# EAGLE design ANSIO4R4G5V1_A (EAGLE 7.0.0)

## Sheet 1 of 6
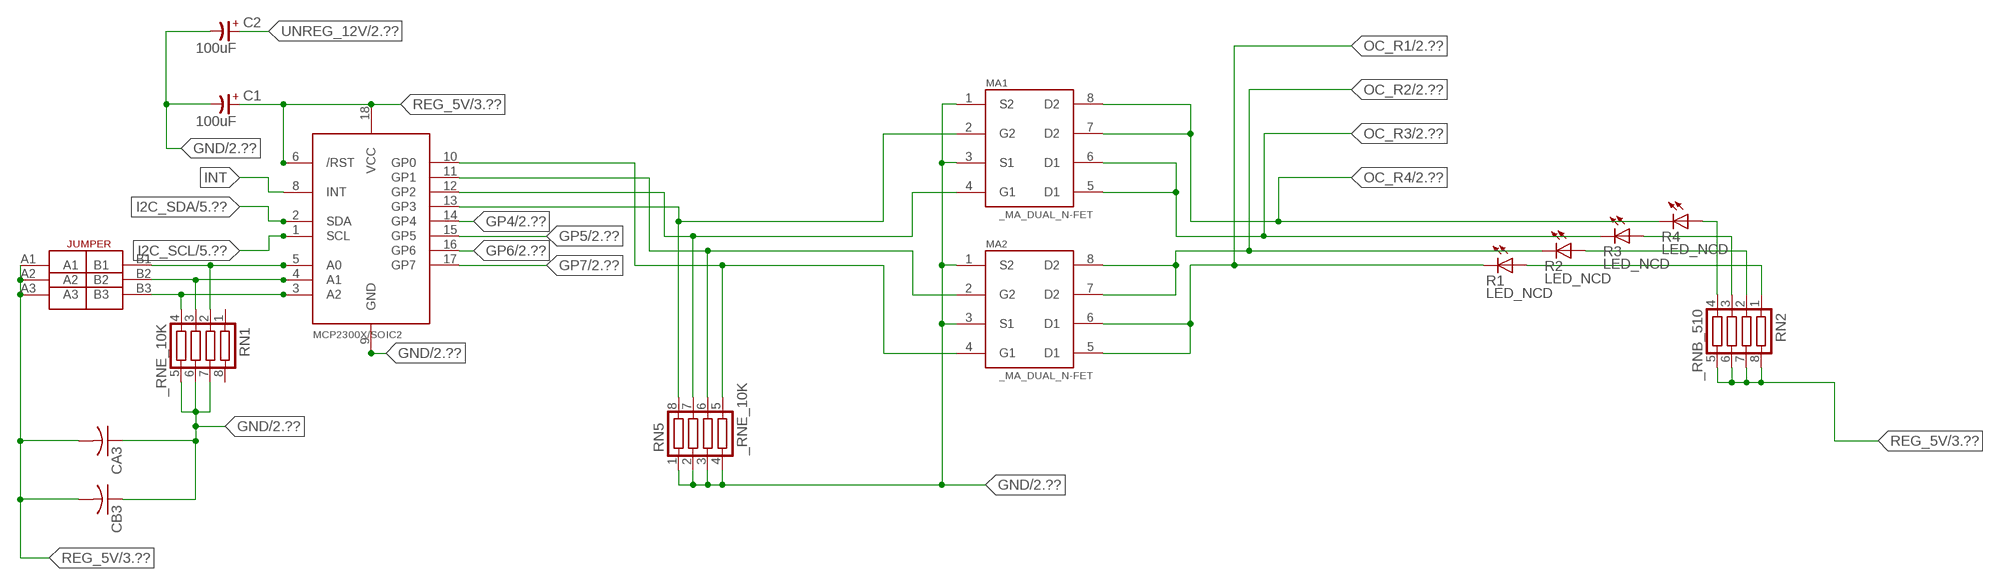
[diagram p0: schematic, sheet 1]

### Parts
C1  100uF  CP-E-025X060  [E-025X060]
C2  100uF  CP-E-025X060  [E-025X060]
CA3  CC1206KRX7R9BB104C1206K  [CC1206KRX7R9BB104]
CB3  TMK316F106ZL-TC1206K  [TMK316F106ZL-T]
IC2  MCP2300X/SO  [SO18W]
MA1  _MA_DUAL_N-FET  [_MA_DUAL_N-FET]
MA2  _MA_DUAL_N-FET  [_MA_DUAL_N-FET]
R1  LED_NCD  [CHIPLED_0603]
R2  LED_NCD  [CHIPLED_0603]
R3  LED_NCD  [CHIPLED_0603]
R4  LED_NCD  [CHIPLED_0603]
RN1  _RNE_10K  [RNE]
RN2  _RNB_510  [RNB]
RN5  _RNE_10K  [RNE]
U$18  JUMPER_3X2  [JUMPER_3X2]

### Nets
GND: C1.- C2.- CA3.1 CB3.1 IC2.9(GND) MA1.1(S2) MA1.3(S1) MA2.1(S2) MA2.3(S1) RN1.5 RN1.6 RN1.7 RN5.1 RN5.2 RN5.3 RN5.4 ; also sheet 2,3,4,5,6
GP4: IC2.14(GP4) ; also sheet 2
GP5: IC2.15(GP5) ; also sheet 2
GP6: IC2.16(GP6) ; also sheet 2
GP7: IC2.17(GP7) ; also sheet 2
I2C_SCL: IC2.1(SCL) ; also sheet 5,6
I2C_SDA: IC2.2(SDA) ; also sheet 5,6
INT: IC2.8(INT)
N$6: IC2.5(A0) RN1.2 U$18.B1
N$7: IC2.4(A1) RN1.3 U$18.B2
N$8: IC2.3(A2) RN1.4 U$18.B3
N$20: IC2.13(GP3) MA1.2(G2) RN5.8
N$21: IC2.12(GP2) MA1.4(G1) RN5.7
N$22: IC2.11(GP1) MA2.2(G2) RN5.6
N$23: IC2.10(GP0) MA2.4(G1) RN5.5
N$29: R4.A RN2.4
N$30: R3.A RN2.3
N$31: R2.A RN2.2
N$32: R1.A RN2.1
OC_R1: MA2.5(D1) MA2.6(D1) R1.C ; also sheet 2
OC_R2: MA2.7(D2) MA2.8(D2) R2.C ; also sheet 2
OC_R3: MA1.5(D1) MA1.6(D1) R3.C ; also sheet 2
OC_R4: MA1.7(D2) MA1.8(D2) R4.C ; also sheet 2
REG_5V: C1.+ CA3.2 CB3.2 IC2.6(/RST) IC2.18(VCC) RN2.5 RN2.6 RN2.7 RN2.8 U$18.A1 U$18.A2 U$18.A3 ; also sheet 3,4,5,6
UNREG_12V: C2.+ ; also sheet 2,3
Unconnected: RN1.1 RN1.8

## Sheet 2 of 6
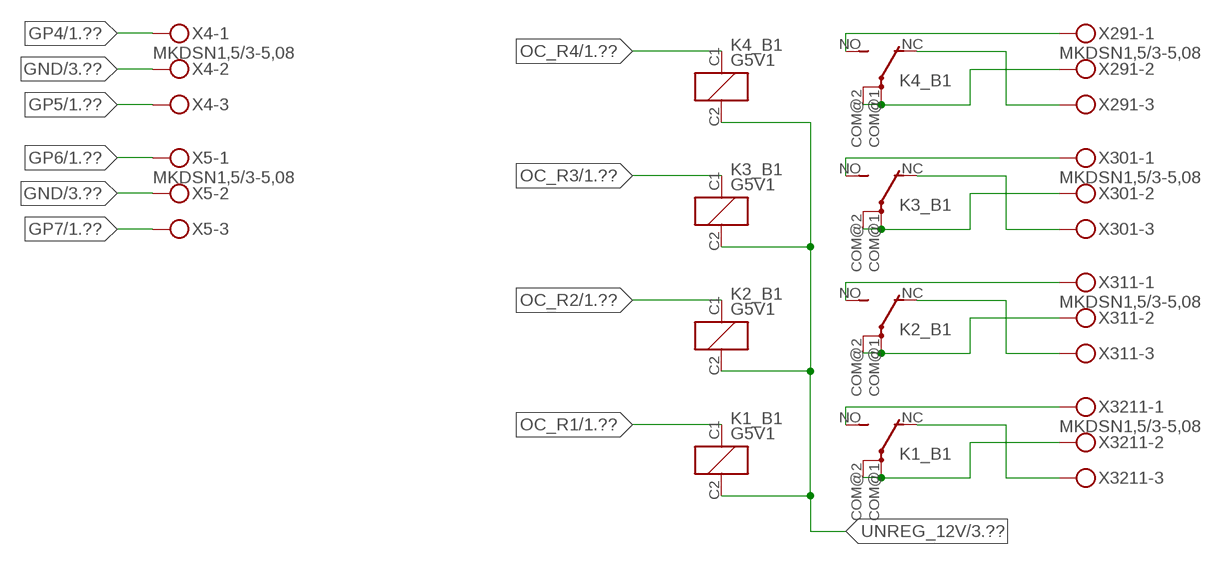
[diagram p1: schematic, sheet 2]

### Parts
K1_B1  G5V1  [G5V1]
K2_B1  G5V1  [G5V1]
K3_B1  G5V1  [G5V1]
K4_B1  G5V1  [G5V1]
X4  MKDSN1,5/3-5,08  [MKDSN1,5/3-5,08]
X5  MKDSN1,5/3-5,08  [MKDSN1,5/3-5,08]
X291  MKDSN1,5/3-5,08  [MKDSN1,5/3-5,08]
X301  MKDSN1,5/3-5,08  [MKDSN1,5/3-5,08]
X311  MKDSN1,5/3-5,08  [MKDSN1,5/3-5,08]
X3211  MKDSN1,5/3-5,08  [MKDSN1,5/3-5,08]

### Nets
GND: X4.2 X5.2 ; also sheet 1,3,4,5,6
GP4: X4.1 ; also sheet 1
GP5: X4.3 ; also sheet 1
GP6: X5.1 ; also sheet 1
GP7: X5.3 ; also sheet 1
N$215: K4_B1.NO(2:S) X291.1
N$216: K4_B1.NC(2:O) X291.3
N$217: K4_B1.COM@1(2:P) K4_B1.COM@2(2:P) X291.2
N$218: K3_B1.NO(2:S) X301.1
N$219: K3_B1.NC(2:O) X301.3
N$220: K3_B1.COM@1(2:P) K3_B1.COM@2(2:P) X301.2
N$221: K2_B1.NO(2:S) X311.1
N$222: K2_B1.NC(2:O) X311.3
N$223: K2_B1.COM@1(2:P) K2_B1.COM@2(2:P) X311.2
N$224: K1_B1.NO(2:S) X3211.1
N$225: K1_B1.NC(2:O) X3211.3
N$226: K1_B1.COM@1(2:P) K1_B1.COM@2(2:P) X3211.2
OC_R1: K1_B1.C1(1:C1) ; also sheet 1
OC_R2: K2_B1.C1(1:C1) ; also sheet 1
OC_R3: K3_B1.C1(1:C1) ; also sheet 1
OC_R4: K4_B1.C1(1:C1) ; also sheet 1
UNREG_12V: K1_B1.C2(1:C2) K2_B1.C2(1:C2) K3_B1.C2(1:C2) K4_B1.C2(1:C2) ; also sheet 1,3

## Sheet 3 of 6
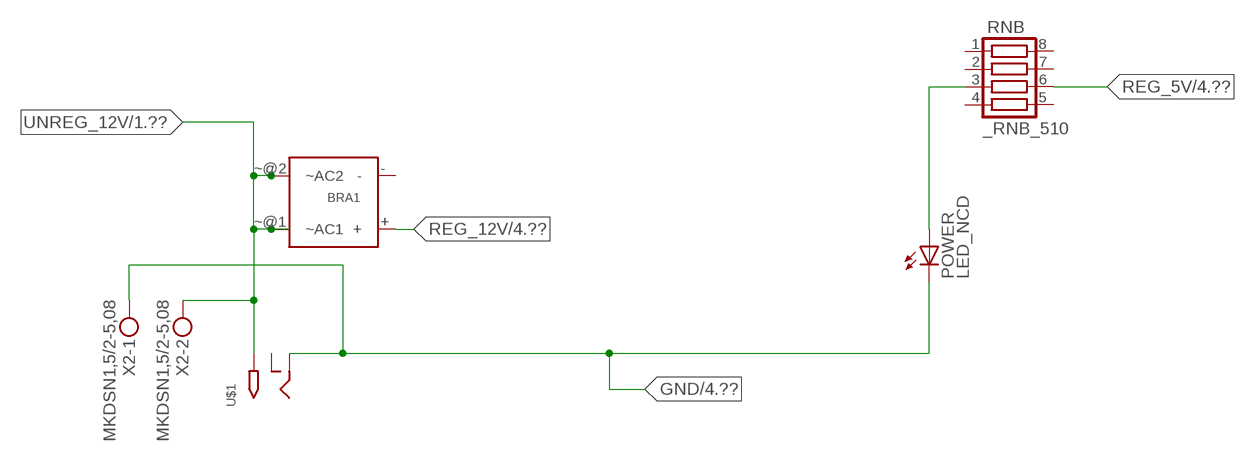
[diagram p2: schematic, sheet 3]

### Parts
BRA1  MB2S_  [MB2S]
POWER  LED_NCD  [CHIPLED_0603]
RNB  _RNB_510  [RNB]
U$1  2.1MMJACK  [PJ-102A]
X2  MKDSN1,5/2-5,08  [MKDSN1,5/2-5,08]

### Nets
GND: POWER.C U$1.RING X2.1 ; also sheet 1,2,4,5,6
N$2: POWER.A RNB.3
REG_5V: RNB.6 ; also sheet 1,4,5,6
REG_12V: BRA1.+ ; also sheet 4
UNREG_12V: BRA1.~@1(~AC1) BRA1.~@2(~AC2) U$1.TIP X2.2 ; also sheet 1,2
Unconnected: BRA1.- RNB.1 RNB.2 RNB.4 RNB.5 RNB.7 RNB.8 U$1.RING_SW

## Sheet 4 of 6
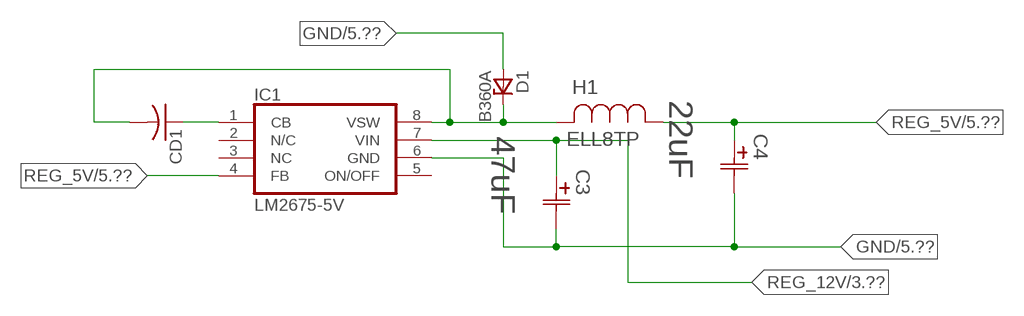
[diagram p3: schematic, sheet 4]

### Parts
C3  47uF  490-5463-6-NDCAP  [C2917(7343)-Y]
C4  22uF  490-5463-6-NDCAP  [C2917(7343)-Y]
CD1  _CD_10NF_50VC1206K  [_CD_10NF_50V]
D1  B360A  [DO214AC_ZENER]
H1  ELL8TP  [IND_ELL8TP]
IC1  LM2675-5V  LM2675  [SO-8]

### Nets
GND: C3.2(C2) C4.2(C2) D1.A IC1.6(GND) ; also sheet 1,2,3,5,6
N$1: CD1.2 D1.C H1.2 IC1.8(VSW)
N$3: CD1.1 IC1.1(CB)
REG_5V: C4.1(C1) H1.1 IC1.4(FB) ; also sheet 1,3,5,6
REG_12V: C3.1(C1) IC1.7(VIN) ; also sheet 3
Unconnected: IC1.2(N/C) IC1.5(ON/OFF)

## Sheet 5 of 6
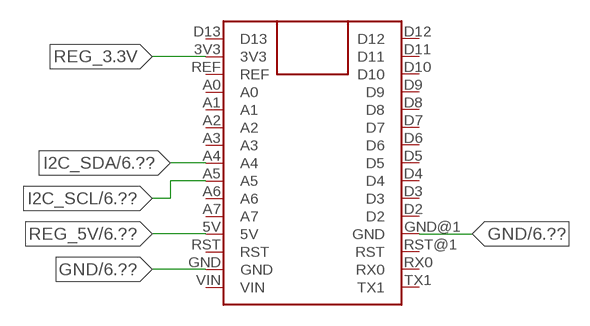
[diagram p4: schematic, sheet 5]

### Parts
FOR_NANO  ARDUINO_NANO  [ARDUINO_NANO]

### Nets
GND: FOR_NANO.GND FOR_NANO.GND@1(GND) ; also sheet 1,2,3,4,6
I2C_SCL: FOR_NANO.A5 ; also sheet 1,6
I2C_SDA: FOR_NANO.A4 ; also sheet 1,6
REG_3.3V: FOR_NANO.3V3
REG_5V: FOR_NANO.5V ; also sheet 1,3,4,6
Unconnected: FOR_NANO.A0 FOR_NANO.A1 FOR_NANO.A2 FOR_NANO.A3 FOR_NANO.A6 FOR_NANO.A7 FOR_NANO.D2 FOR_NANO.D3 FOR_NANO.D4 FOR_NANO.D5 FOR_NANO.D6 FOR_NANO.D7 FOR_NANO.D8 FOR_NANO.D9 FOR_NANO.D10 FOR_NANO.D11 FOR_NANO.D12 FOR_NANO.D13 FOR_NANO.REF FOR_NANO.RST FOR_NANO.RST@1(RST) FOR_NANO.RX0 FOR_NANO.TX1 FOR_NANO.VIN

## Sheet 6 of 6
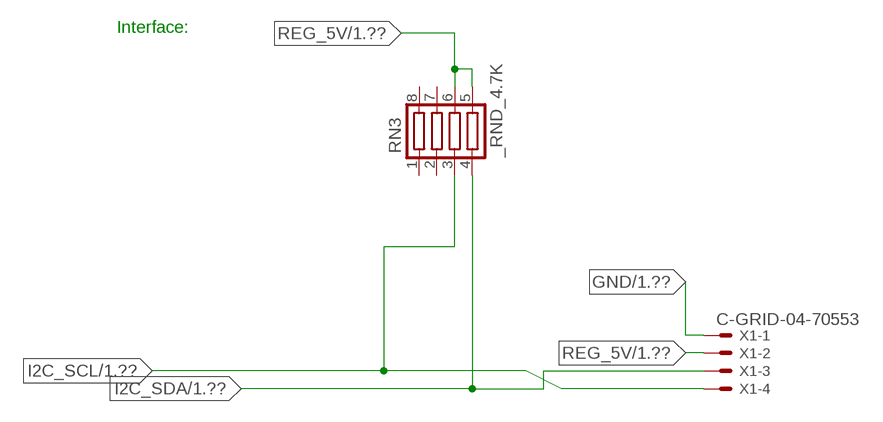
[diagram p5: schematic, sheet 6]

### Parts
RN3  _RND_4.7K  [RND]
X1  C-GRID-04-70553  [70553-04]

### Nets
GND: X1.1 ; also sheet 1,2,3,4,5
I2C_SCL: RN3.3 X1.4 ; also sheet 1,5
I2C_SDA: RN3.4 X1.3 ; also sheet 1,5
REG_5V: RN3.5 RN3.6 X1.2 ; also sheet 1,3,4,5
Unconnected: RN3.1 RN3.2 RN3.7 RN3.8

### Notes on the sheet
- Interface:

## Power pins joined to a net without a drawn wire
NC: IC1.3(NC)

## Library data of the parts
BRA1 = NCD_ULTIMATE_LIBRARY:MB2S: Bridge Rectifier BRA MB2S 200V 500ma Digikey MB2S-TPMSTR-ND/MB2S-TP
C1 C2 = NCD_ULTIMATE_LIBRARY:CP-: Capacitors All Kinds POLARIZED CAP
C3 C4 = NCD_ULTIMATE_bhaskar:490-5463-6-ND: NCD CAP
CA3 = NCD_ULTIMATE_LIBRARY:CC1206KRX7R9BB104: Capacitor CA .1uF 50V SMT C1206K CC1206KRX7R9BB104
CB3 = NCD_ULTIMATE_LIBRARY:TMK316F106ZL-T: Capacitor CB 10uF SMT 1206 TMK316F106ZL-T
CD1 = NCD_ULTIMATE_LIBRARY:_CD_10NF_50V: Capacitor 10nF SMT
D1 = NCD_ULTIMATE_bhaskar:B360A: NCD DIODE B350A/B360A
FOR_NANO = NCD_ULTIMATE_CONNECTORS:ARDUINO_NANO
H1 = NCD_ULTIMATE_bhaskar:ELL8TP: NCD coil
IC1 = NCD_ULTIMATE_bhaskar:LM2675: LM2675 NCD http://www.ti.com/lit/ds/symlink/lm2675.pdf
IC2 = NCD_ULTIMATE_LIBRARY:MCP2300X: Semiconductor Port Expander I/O 8-Bit I2C MCP23008 Inexpensive i2c i/o expander - 8 general purpose i/o pins with optional pullups
K1_B1 K2_B1 K3_B1 K4_B1 = NCD_ULTIMATE_LIBRARY:G5V1: RELAY 1 x switch, 0.5 A/125 V AC, 1 A/24 V DC , Omron
MA1 MA2 = NCD_ULTIMATE_LIBRARY:_MA_DUAL_N-FET: FET Dual N-Channel 8-SOIC NMOSFET Digikey 785-1064-2-ND/AO4842
POWER = NCD_ULTIMATE_bhaskar:LED_NCD
R1-R4 = NCD_ULTIMATE_LIBRARY:LED_NCD: LED Digikey 754-1132-2-ND/APT2012SRCPRV
RN1 RN5 = NCD_ULTIMATE_LIBRARY:_RNE_10K: Resistor Array RNE SMT 10K x 4 Single Resistor Source: http://www.ctscorp.com/components/Datasheets/CTSChipArrayDs.pdf Digikey 742C083103JPTR-ND/742C083103JP; OC_FARNELL: unknown; OC_NEWARK: unknown
RN2 RNB = NCD_ULTIMATE_LIBRARY:_RNB_510: Resistor Array RNB SMT 510 x 4 Single Resistor Source: http://www.ctscorp.com/components/Datasheets/CTSChipArrayDs.pdf Digikey 742C083511JPTR-ND/ 742C083511JP; OC_FARNELL: unknown; OC_NEWARK: unknown
RN3 = NCD_ULTIMATE_LIBRARY:_RND_4.7K: Resistor Array RND SMT 4.7K x 4 Single Resistor Source: http://www.ctscorp.com/components/Datasheets/CTSChipArrayDs.pdf Digikey 742C083472JPTR-ND/742C083472JP; OC_FARNELL: unknown; OC_NEWARK: unknown
U$1 = NCD_ULTIMATE_CONNECTORS:2.1MMJACK: 2.1mm x 5.5mm DC jack with internal switch. Digikey part #PJ-102A, 4UCON part #05537 By microbuilder.eu
U$18 = NCD_ULTIMATE_CONNECTORS:JUMPER_3X2
X1 = NCD_ULTIMATE_CONNECTORS:C-GRID-04: CONNECTOR 4-Pos I2C wire to board 2.54 mm (0.100") pitch header Digikey WM1342-ND/0015912045; OC_FARNELL: unknown; OC_NEWARK: unknown
X2 = NCD_ULTIMATE_CONNECTORS:MKDSN1,5/2-5,08: MKDSN 1,5/ 2-5,08 Printklemme
X4 X5 X291 X301 X311 X3211 = NCD_ULTIMATE_CONNECTORS:MKDSN1,5/3-5,08: MKDSN 1,5/ 3-5,08 Printklemme Nennstrom: 13,5 A Nennspannung: 250 V Rastermaß: 5,08 mm Polzahl: 3 Anschlussart: Schraubanschluss Montage: Löten Anschlussrichtung Leiter/Platine: 0 ° Artikelnummer: 1729131 Source: http://eshop.phoenixcontact.com .. 1729131.pdf

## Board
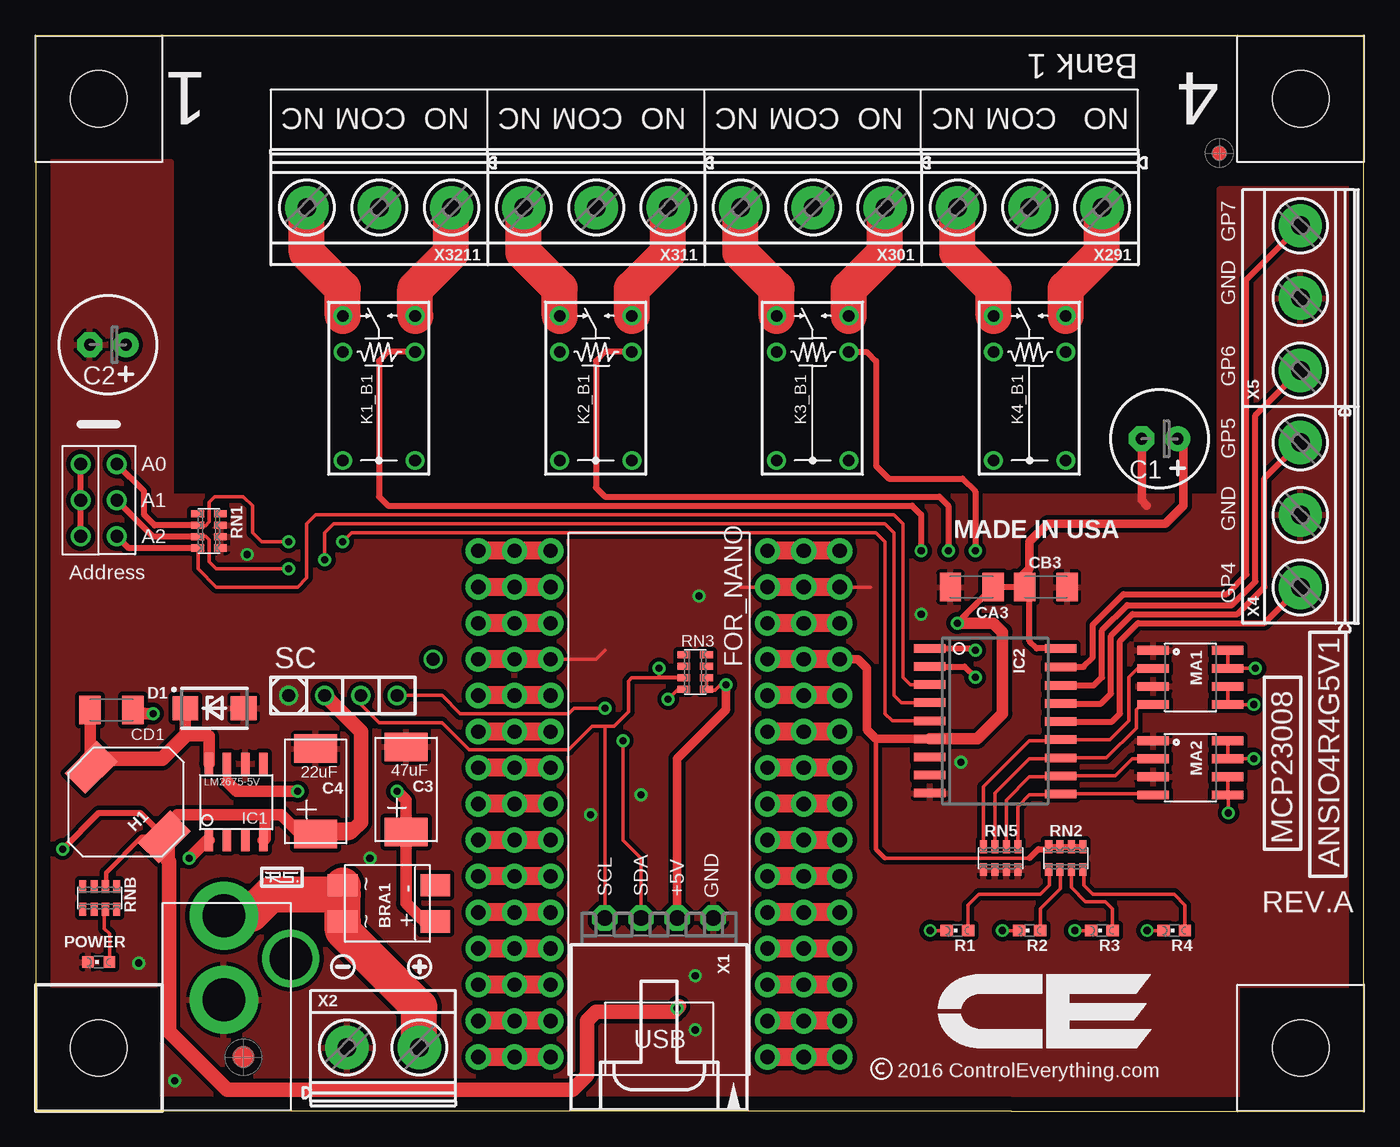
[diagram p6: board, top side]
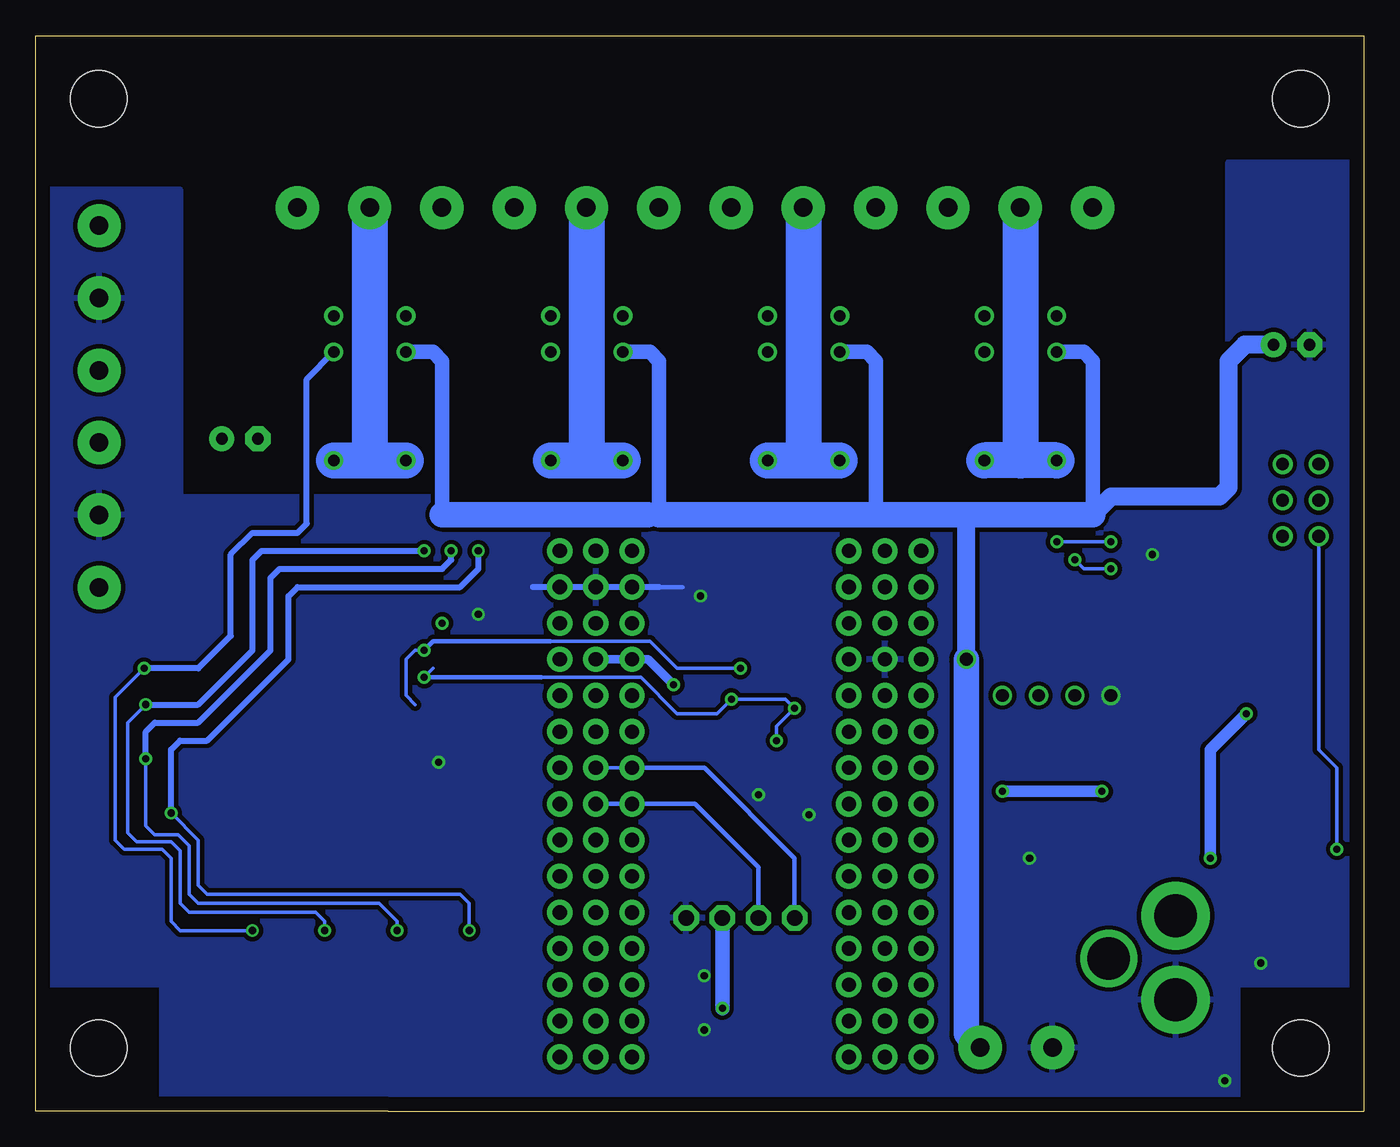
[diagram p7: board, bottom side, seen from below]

Size 93.34 x 75.56 mm. Coordinates in mm from the lower left corner, seen from the top.
Outline: 0,56.19 0,55.24
Outline: 0,55.24 0,0 68.58,0 93.34,0 93.34,75.56 0,75.56 0,55.24
Copper layers (1*16): Top 0.035mm / dielectric 1.5mm / Bottom 0.035mm
Design rules "default": minimum track width 10mil, minimum drill 24mil, track to track 8mil, track to pad 8mil, pad to pad 8mil, via to via 8mil, smd to smd 8mil, copper to edge 40mil, drill to drill 8mil, minimum pad ring 10mil, minimum via ring 8mil, stop-mask expansion 4mil, vias tented up to drill 0mil, thermal gap 10mil
Holes 3.96 mm at 4.45,4.45 4.45,4.45 4.45,4.45

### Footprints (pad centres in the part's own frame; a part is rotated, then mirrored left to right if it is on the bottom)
MB2S = smd 1.55 x 2.1: + 0,-6.5; - 2.54,-6.5; ~@1 0,0; ~@2 2.54,0
E-025X060 = drill 0.813 pad 1.778: + -1.27,0 | drill 0.813 pad 1.778 octagon: - 1.27,0
C2917(7343)-Y = smd 2 x 3: 1 -3,0; 2 3,0
CC1206KRX7R9BB104 = smd 1.5 x 2: 1 -1.5,0; 2 1.5,0
TMK316F106ZL-T = smd 1.5 x 2: 1 -1.5,0; 2 1.5,0
_CD_10NF_50V = smd 1.5 x 2: 1 -1.5,0; 2 1.5,0
DO214AC_ZENER = smd 1.8 x 1.7: A 2.05,0; C -2.05,0
ARDUINO_NANO = drill 1 pad 1.778: 3V1 -2.54,-2.54; 3V3 0,-2.54; 5V 0,-27.94; 5V1 -2.54,-27.94; A0 0,-7.62; A1 0,-10.16; A2 0,-12.7; A3 0,-15.24; A4 0,-17.78; A5 0,-20.32; A6 0,-22.86; A7 0,-25.4; A8 -2.54,-7.62; A9 -2.54,-10.16; A10 -2.54,-12.7; A11 -2.54,-15.24; A12 -2.54,-17.78; A13 -2.54,-20.32; A14 -2.54,-22.86; A15 -2.54,-25.4; D1 -2.54,0; D2 20.32,-25.4; D3 20.32,-22.86; D4 20.32,-20.32; D5 20.32,-17.78; D6 20.32,-15.24; D7 20.32,-12.7; D8 20.32,-10.16; D9 20.32,-7.62; D10 20.32,-5.08; D11 20.32,-2.54; D12 20.32,0; D13 0,0; D14 22.86,0; D15 22.86,-2.54; D16 22.86,-5.08; D17 22.86,-7.62; D18 22.86,-10.16; D19 22.86,-12.7; D20 22.86,-15.24; D21 22.86,-17.78; D22 22.86,-20.32; D23 22.86,-22.86; D24 22.86,-25.4; GND 0,-33.02; GND1 -2.54,-33.02; GND@1 20.32,-27.94; GND@2 22.86,-27.94; P$16 2.54,0; P$17 2.54,-2.54; P$18 2.54,-5.08; P$19 2.54,-7.62; P$20 2.54,-10.16; P$21 2.54,-12.7; P$22 2.54,-15.24; P$23 2.54,-17.78; P$24 2.54,-20.32; P$25 2.54,-22.86; P$26 2.54,-25.4; P$27 2.54,-27.94; P$28 2.54,-30.48; P$29 2.54,-33.02; P$30 2.54,-35.56; P$31 17.78,0; P$32 17.78,-2.54; P$33 17.78,-5.08; P$34 17.78,-7.62; P$35 17.78,-10.16; P$36 17.78,-12.7; P$37 17.78,-15.24; P$38 17.78,-17.78; P$39 17.78,-20.32; P$40 17.78,-22.86; P$41 17.78,-25.4; P$42 17.78,-27.94; P$43 17.78,-30.48; P$44 17.78,-33.02; P$45 17.78,-35.56; REF 0,-5.08; REF1 -2.54,-5.08; RST 0,-30.48; RST1 -2.54,-30.48; RST@1 20.32,-30.48; RST@2 22.86,-30.48; RX0 20.32,-33.02; RX1 22.86,-33.02; TX1 20.32,-35.56; TX2 22.86,-35.56; VIN 0,-35.56; VIN1 -2.54,-35.56
IND_ELL8TP = smd 2.054 x 3.2 rotated 45: 1 -2.442,-2.696; 2 2.442,2.442
SO-8 = smd 0.6 x 1.55: 1 -1.905,-2.69; 2 -0.635,-2.69; 3 0.635,-2.69; 4 1.905,-2.69; 5 1.905,2.71; 6 0.635,2.71; 7 -0.635,2.71; 8 -1.905,2.71
SO18W = smd 0.6 x 2.2: 1 -4.445,-4.6; 2 -3.175,-4.6; 3 -1.905,-4.6; 4 -0.635,-4.6; 5 0.635,-4.6; 6 1.905,-4.6; 7 3.175,-4.6; 8 4.445,-4.6; 9 5.715,-4.6; 10 5.775,4.6; 11 4.505,4.6; 12 3.235,4.6; 13 1.965,4.6; 14 0.695,4.6; 15 -0.575,4.6; 16 -1.845,4.6; 17 -3.145,4.6; 18 -4.445,4.6
G5V1 = drill 0.813: C1 -2.54,2.54; C2 -2.54,-2.54; COM@1 5.08,-2.54; COM@2 5.08,2.54; NC -5.08,-2.54; NO -5.08,2.54
_MA_DUAL_N-FET = smd 0.61 x 2.21: 1 -1.905,-2.616; 2 -0.635,-2.616; 3 0.635,-2.616; 4 1.905,-2.616; 5 1.905,2.616; 6 0.635,2.616; 7 -0.635,2.616; 8 -1.905,2.616
CHIPLED_0603 = smd 0.8 x 0.8: A 0,-0.75; C 0,0.75
CHIPLED_0603' = smd 0.8 x 0.876: A 0,-0.75; C 0,0.75
RNE = smd 0.5 x 0.9: 1 -1.2,-0.8; 2 -0.4,-0.8; 3 0.4,-0.8; 4 1.2,-0.8; 5 1.2,0.8; 6 0.4,0.8; 7 -0.4,0.8; 8 -1.2,0.8
RNB = smd 0.5 x 0.9: 1 -1.2,-0.8; 2 -0.4,-0.8; 3 0.4,-0.8; 4 1.2,-0.8; 5 1.2,0.8; 6 0.4,0.8; 7 -0.4,0.8; 8 -1.2,0.8
RND = smd 0.5 x 0.9: 1 -1.2,-0.8; 2 -0.4,-0.8; 3 0.4,-0.8; 4 1.2,-0.8; 5 1.2,0.8; 6 0.4,0.8; 7 -0.4,0.8; 8 -1.2,0.8
PJ-102A = drill 3 pad 4.8: RING 0.1,-3.39; TIP 0.1,-9.29 | drill 3 pad 3.251: RING_SW -4.6,-6.29
PCB_MOUNTING_HOLE = hole 3.962: 4.445,4.445
JUMPER_3X2 = drill 0.9: A1 0,5.08; A2 0,2.54; A3 0,0; B1 2.54,5.08; B2 2.54,2.54; B3 2.54,0
70553-04 = drill 1.1 pad 1.778 octagon: 1 -3.81,-7.62; 2 -1.27,-7.62; 3 1.27,-7.62; 4 3.81,-7.62
MKDSN1,5/2-5,08 = drill 1.3 pad 3.048: 1 -2.561,0.025; 2 2.519,0.025
MKDSN1,5/3-5,08 = drill 1.3 pad 3.048: 1 -7.641,0.025; 2 -2.561,0.025; 3 2.519,0.025

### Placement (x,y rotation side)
BRA1  21.59,13.34 90 top
C1  78.99,47.24 180 top
C2  5.08,53.85 180 top
C3  26.04,22.61 90 top
C4  19.68,22.48 90 top
CA3  65.79,36.83 0 top
CB3  70.99,36.83 180 top
CD1  5.33,28.19 180 top
D1  12.57,28.32 0 top
FOR_NANO  53.98,3.81 180 top
H1  6.35,21.72 90 top
IC1  14.1,21.72 0 top
IC2  67.44,28.07 270 top
K1_B1  24.13,50.8 270 top
K2_B1  39.37,50.8 270 top
K3_B1  54.61,50.8 270 top
K4_B1  69.85,50.8 270 top
MA1  81.15,30.48 270 top
MA2  81.15,24.13 270 top
POWER  4.45,10.48 90 top
R1  LED_NCD  [CHIPLED_0603']  64.77,12.7 90 top
R2  LED_NCD  [CHIPLED_0603']  69.85,12.7 90 top
R3  LED_NCD  [CHIPLED_0603']  74.93,12.7 90 top
R4  LED_NCD  [CHIPLED_0603']  80.01,12.7 90 top
RN1  12.19,40.77 270 top
RN2  72.39,17.78 0 top
RN3  46.35,30.86 270 top
RN5  67.82,17.78 0 top
RNB  4.51,14.99 0 top
U$1  13.34,4.45 180 top
U$2  [VISION_REF15]  14.61,3.81 0 top
U$3  [ICON_MINUS]  21.59,10.16 180 top
U$4  PCB_MOUNTING_HOLE  [PCB_MOUNTING_HOLE]  93.34,66.67 90 top
U$5  [ICON_PLUS]  26.99,10.16 90 top
U$6  PCB_MOUNTING_HOLE  [PCB_MOUNTING_HOLE]  93.34,0 90 top
U$11  PCB_MOUNTING_HOLE  [PCB_MOUNTING_HOLE]  8.89,66.67 90 top
U$18  3.17,40.39 0 top
U$19  [VISION_REF10]  83.19,67.31 0 top
U$21  [ICON_USA]  64.52,40.26 0 top
X1  43.81,5.97 180 top
X2  24.45,4.45 0 top
X4  88.9,44.45 90 top
X5  88.9,59.69 90 top
X291  67.31,63.5 180 top
X301  52.07,63.5 180 top
X311  36.83,63.5 180 top
X3211  21.59,63.5 180 top

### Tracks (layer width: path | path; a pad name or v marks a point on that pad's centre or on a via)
GND  (via drill 0.5, 0.9)
  Top 0.254: 36.2,31.75 39.37,31.75 40.01,32.39 | FOR_NANO.GND@1 32.38,31.75 | 49.53,36.83 56.52,36.83 58.67,36.83
  Top 0.61: C1.- 77.72,42.93 78.11,42.55
  Top 1.016: X1.1 47.62,13.74
  Bottom 0.254: 51.44,36.83 FOR_NANO.GND
  Bottom 0.305: 47.88,36.83 49.53,36.83 51.44,36.83
  Bottom 0.406: 49.53,36.83 58.42,36.83
  other vias: 14.86,39.12 65.02,24.51 62.23,34.92 9.78,2.16 17.78,29.21 46.35,9.53 46.61,36.2 46.35,5.72 42.55,22.23 38.99,20.83 7.24,10.41 23.5,17.78
  pour Bottom (isolate 0.305): -1.91,8.89 8.89,8.89 8.89,0 84.45,0 84.45,8.89 92.71,8.89 92.71,64.77 83.19,64.77 83.19,43.18 9.53,43.18 9.53,66.67 -1.91,66.67
  pour Top (isolate 0.305): -3.81,8.89 8.89,8.89 8.89,0 84.45,0 84.45,8.89 92.71,8.89 92.71,64.77 83.19,64.77 83.19,43.18 9.53,43.18 9.53,66.67 -3.81,66.67
GP4
  Top 0.406: IC2.14 75.63,27.37 76.2,27.94 76.2,33.02 77.47,34.29 86.36,34.29 X4.1
GP5
  Top 0.406: IC2.15 74.87,28.64 75.56,29.34 75.56,33.4 77.09,34.92 84.45,34.92 86.36,36.83 86.36,44.45 X4.3
GP6
  Top 0.406: IC2.16 74.36,29.91 74.93,30.48 74.93,33.78 76.71,35.56 84.07,35.56 85.72,37.21 85.72,48.9 X5.1
GP7
  Top 0.406: IC2.17 73.63,31.21 74.3,31.88 74.3,34.16 76.45,36.32 83.69,36.32 85.09,37.72 85.09,58.42 X5.3
I2C_SCL  (via drill 0.5, 0.9)
  Top 0.254: 40.01,27.05 40.64,27.05 41.66,28.07 41.66,30.23 41.89,30.46 RN3.3 45.54,30.48 43.81,30.48 v43.81,31.12 | 40.01,27.05 39.12,27.05 37.47,25.4 30.48,25.4 28.57,27.3 24.13,27.3 22.86,28.57 v22.86,29.21 | X1.4 40.01,27.05
  Top 0.406: IC2.1 65.91,32.51 v66.04,32.39
  Bottom 0.254: 66.67,28.57 67.31,29.21 67.31,31.75 66.67,32.39 v66.04,32.39 | 57.15,33.02 50.16,33.02 48.26,31.12 v43.81,31.12 | 51.44,24.13 FOR_NANO.A5
  Bottom 0.305: 57.15,33.02 65.41,33.02 v66.04,32.39 | 51.44,24.13 46.35,24.13 40.01,17.78 X1.4
I2C_SDA  (via drill 0.5, 0.9)
  Top 0.254: RN3.4 45.16,29.66 v44.45,28.96 | 40,28.33 v40.01,28.32 37.85,28.32 37.47,27.94 29.84,27.94 28.57,29.21 v25.4,29.21 | X1.3 42.55,17.78 41.27,19.05 v41.27,26.04
  Top 0.406: IC2.2 65.28,31.24 v66.04,30.48
  Bottom 0.254: 65.41,31.12 v66.04,30.48 | v41.27,26.04 41.27,27.05 v40.01,28.32 40.64,28.96 v44.45,28.96 45.47,27.94 48.26,27.94 50.8,30.48 57.78,30.48
  Bottom 0.305: 57.78,30.48 v66.04,30.48 | FOR_NANO.A4 46.99,21.59 42.55,17.15 X1.3
N$1
  Top 0.813: H1.2 3.88,24.77 | D1.C 10.52,26.4 12.19,26.38 IC1.8 | CD1.2 3.83,24.15 4.45,24.77
  Top 1.016: 3.88,24.77 4.45,24.77 8.89,24.77 10.52,26.4
N$2
  Top 0.254: POWER.A 5.2,12.46 4.83,12.83 4.83,14.1 RNB.3
  Top 0.406: 4.95,14.14 RNB.3
N$3  (via drill 0.5)
  Top 0.813: IC1.1 12.04,19.03 v10.79,17.78 | v8.26,27.94 7.72,27.94 CD1.1
  Bottom 0.813: v10.79,17.78 10.79,25.4 v8.26,27.94
N$6  (via drill 0.5)
  Top 0.254: IC2.5 60.2,27.43 59.69,27.94 59.69,40 59.05,40.64 22.23,40.64 v21.59,40 | v17.78,40 15.88,40 15.24,40.64 15.24,42.55 14.61,43.18 12.57,43.18 12.19,42.8 12.19,41.4 11.94,41.15 11.41,41.15 RN1.2
  Top 0.406: RN1.2 8.36,41.17 7.62,41.91 7.62,43.56 U$18.B1
  Bottom 0.254: v21.59,40 v17.78,40
N$7  (via drill 0.5)
  Top 0.254: IC2.4 60.83,28.7 60.33,29.21 60.33,40.64 59.69,41.27 20.95,41.27 20.32,40.64 v20.32,38.73 | v17.78,38.1 12.7,38.1 12.19,38.61 12.19,40.13 11.94,40.39 11.41,40.39 RN1.3
  Top 0.406: RN1.3 8.27,40.37 U$18.B2
  Bottom 0.254: v20.32,38.73 19.68,38.1 v17.78,38.1
N$8
  Top 0.254: IC2.3 61.47,29.97 60.96,30.48 60.96,41.27 60.33,41.91 19.68,41.91 19.05,41.27 19.05,37.47 18.41,36.83 12.7,36.83 11.43,38.1 11.43,39.53 RN1.4
  Top 0.406: RN1.4 6.53,39.57 U$18.B3
N$20
  Top 0.254: MA1.2 77.47,31.12 76.83,30.48 76.83,27.43 75.5,26.1 IC2.13 71.97,26.04 69.85,26.04 66.62,22.8 RN5.8
N$21
  Top 0.254: MA1.4 77.72,28.57 77.34,28.19 77.34,26.92 75.25,24.83 IC2.12 71.97,24.77 69.85,24.77 67.42,22.33 RN5.7
N$22
  Top 0.254: MA2.2 77.09,24.77 75.89,23.56 IC2.11 71.97,23.5 69.85,23.5 68.22,21.86 RN5.6
N$23
  Top 0.254: MA2.4 78.6,22.29 IC2.10 71.97,22.23 69.85,22.23 69.02,21.39 RN5.5
N$29
  Top 0.254: R4.A 80.76,14.49 80.01,15.24 74.3,15.24 73.66,15.88 73.66,16.91 RN2.4
N$30
  Top 0.254: R3.A 75.68,14.24 75.18,14.73 73.79,14.73 72.77,15.75 72.77,16.96 RN2.3
N$31
  Top 0.254: R2.A 70.6,14.21 72.01,15.62 72.01,16.96 RN2.2
N$32
  Top 0.254: R1.A 65.52,14.47 66.29,15.24 70.61,15.24 71.25,15.88 71.25,16.92 RN2.1
N$215
  Top 2.54: K4_B1.NO 72.39,57.79 74.93,60.33 74.93,63.45 X291.1
N$216
  Top 2.54: K4_B1.NC 67.31,57.79 64.77,60.33 64.77,63.45 X291.3
N$217
  Bottom 2.54: X291.2 69.87,45.74 | 69.87,45.74 69.85,45.72 K4_B1.COM@1 | K4_B1.COM@2 69.89,45.72 69.87,45.74
N$218
  Top 2.54: K3_B1.NO 57.15,57.79 59.69,60.33 59.69,63.45 X301.1
N$219
  Top 2.54: K3_B1.NC 52.07,57.79 49.53,60.33 49.53,63.45 X301.3
N$220
  Bottom 2.54: K3_B1.COM@2 54.61,45.72 | 54.61,45.72 K3_B1.COM@1 | X301.2 54.63,45.74 54.61,45.72
N$221
  Top 2.54: K2_B1.NO 41.91,57.79 44.45,60.33 44.45,63.45 X311.1
N$222
  Top 2.54: K2_B1.NC 36.83,57.79 34.29,60.33 34.29,63.45 X311.3
N$223
  Bottom 2.54: K2_B1.COM@2 39.37,45.72 | 39.37,45.72 K2_B1.COM@1 | X311.2 39.39,45.74 39.37,45.72
N$224
  Top 2.54: K1_B1.NO 26.67,57.79 29.21,60.33 29.21,63.45 X3211.1
N$225
  Top 2.54: K1_B1.NC 21.59,57.79 19.05,60.33 19.05,63.45 X3211.3
N$226
  Bottom 2.54: K1_B1.COM@1 24.13,45.72 | 24.13,45.72 K1_B1.COM@2 | X3211.2 24.15,45.74 24.13,45.72
OC_R1  (via drill 0.5)
  Top 0.254: R1.C v62.87,12.7 | v83.82,20.95 83.82,22.15 MA2.5 MA2.6
  Top 0.406: v62.23,39.37 62.23,41.91 61.59,42.55 24.77,42.55 24.13,43.18 24.13,52.7 24.77,53.34 K1_B1.C1
  Bottom 0.254: v62.87,12.7 62.87,14.61 63.5,15.24 81.28,15.24 81.92,15.88 81.92,19.05 v83.82,20.95
  Bottom 0.406: v83.82,20.95 83.82,25.4 83.19,26.04 81.28,26.04 75.56,31.75 75.56,36.2 74.93,36.83 63.5,36.83 62.23,38.1 v62.23,39.37
OC_R2  (via drill 0.5)
  Top 0.254: R2.C v67.94,12.7 | v85.6,24.77 MA2.7 MA2.8
  Top 0.406: v64.14,39.37 64.14,42.55 63.5,43.18 40.01,43.18 39.37,43.81 39.37,52.7 40.01,53.34 K2_B1.C1
  Bottom 0.254: v67.94,12.7 67.94,13.34 69.22,14.61 81.92,14.61 82.55,15.24 82.55,18.67 83.31,19.43 84.96,19.43 85.6,20.07 v85.6,24.77
  Bottom 0.406: v85.6,24.77 85.6,26.67 84.96,27.3 81.92,27.3 76.83,32.39 76.83,37.47 76.2,38.1 64.77,38.1 64.14,38.73 v64.14,39.37
OC_R3  (via drill 0.5)
  Top 0.254: R3.C v73.03,12.7 | v85.6,28.57 MA1.5 MA1.6
  Top 0.406: K3_B1.C1 58.42,53.34 59.05,52.7 59.05,45.35 59.95,44.45 65.14,44.45 66.04,43.55 v66.04,39.37
  Bottom 0.254: v73.03,12.7 73.03,13.34 73.66,13.97 82.55,13.97 83.19,14.61 83.19,18.29 83.82,18.92 86.23,18.92 86.87,19.56 86.87,27.3 v85.6,28.57
  Bottom 0.406: v85.6,28.57 81.92,28.57 78.11,32.39 78.11,38.73 77.47,39.37 v66.04,39.37
OC_R4  (via drill 0.5)
  Top 0.254: R4.C v78.11,12.7 | v85.72,31.12 MA1.7 MA1.8
  Bottom 0.254: v78.11,12.7 83.19,12.7 83.82,13.34 83.82,17.78 84.45,18.41 87.12,18.41 87.76,19.05 87.76,29.08 v85.72,31.12
  Bottom 0.406: v85.72,31.12 81.92,31.12 79.63,33.4 79.63,39.12 78.11,40.64 74.93,40.64 74.3,41.27 74.3,51.44 K4_B1.C1
REG_5V  (via drill 0.5, 0.9)
  Top 0.229: 59.69,17.78 69.85,17.78
  Top 0.254: RN3.6 RN3.5 47.23,29.59 47.75,29.59 48.13,29.97 v48.51,29.97
  Top 0.305: H1.1 7.46,19.27 4.95,16.76 4.95,15.83 RNB.6 | 59.69,17.78 59.05,18.41 59.05,26.16
  Top 0.406: U$18.A3 U$18.A2 U$18.A1 | IC2.18 70.36,32.51 69.85,33.02 69.85,36.47 CB3.2 CA3.2 65.38,34.9 v64.77,34.29 | 62.71,26.04 IC2.6 | 69.85,17.78 70.48,18.41 71.03,18.41 RN2.8 RN2.7 RN2.6 RN2.5 | v1.91,18.41 4.45,20.95 7.37,20.95 H1.1
  Top 0.61: CB3.2 69.22,37.11 69.22,37.47 69.85,38.1 69.85,40 71.12,41.27 79.38,41.27 80.64,42.55 80.64,46.86 C1.+ | FOR_NANO.5V 57.78,31.75 58.42,31.12 58.42,26.8 59.05,26.16 IC2.6 | v48.51,29.97 48.51,28.19 45.09,24.77 X1.2
  Top 0.813: IC2.6 66.17,26.16 67.94,27.94 67.94,33.66 67.31,34.29 v64.77,34.29 | 16.13,20.83 9.96,20.83 H1.1 | 16.13,20.83 17.27,20.83 18.41,19.69 20.75,19.69 C4.1 | IC1.4 16.13,19.15 16.13,20.83
  Top 1.016: H1.1 9.27,18.41 9.27,17.65 9.4,17.53 9.4,5.59 13.46,1.52 37.72,1.52 38.73,2.54 38.73,6.35 39.37,6.99 44.83,6.99 v45.09,7.24 45.21,7.37 | 22.05,19.69 22.23,19.69 22.86,20.32 22.86,26.67 v20.32,29.21
  Top 1.27: 20.75,19.69 22.05,19.69
  Bottom 0.254: U$18.A3 3.17,25.4 1.91,24.13 v1.91,18.41
  Bottom 0.61: FOR_NANO.5V 50.29,31.75 v48.51,29.97
  Bottom 1.016: v45.09,7.24 X1.2
REG_12V  (via drill 0.5)
  Top 0.61: IC1.7 13.46,23.16 | 14.1,22.48 14.15,22.48
  Top 0.813: v18.41,22.48 14.15,22.48 13.46,23.16 | v25.4,22.48 26.04,21.84 C3.1 26.04,14.61 27.3,13.34 BRA1.+
  Bottom 0.813: v18.41,22.48 v25.4,22.48
UNREG_12V  (via drill 0.9)
  Top 2.54: X2.2 26.97,7.32 21.59,12.7 BRA1.~@1 21.59,15.24 | 21.59,15.24 BRA1.~@2 | U$1.TIP 15.14,13.87 16.51,15.24 21.59,15.24
  Bottom 1.016: K4_B1.C2 65.41,53.34 64.77,52.7 64.77,41.91 | K3_B1.C2 50.16,53.34 49.53,52.7 49.53,42.04 | 49.53,42.04 50.29,41.91 | 49.53,42.04 49.66,42.04 49.53,41.91 | K2_B1.C2 34.92,53.34 34.29,52.7 34.29,41.91 | K1_B1.C2 19.68,53.34 19.05,52.7 19.05,41.91
  Bottom 1.27: C2.+ 8.38,53.85 9.53,52.7 9.53,43.81 10.16,43.18 17.78,43.18 19.05,41.91 | v27.94,31.75 27.94,41.91
  Bottom 1.778: 49.53,41.91 34.29,41.91 27.94,41.91 19.05,41.91 | 64.77,41.91 50.29,41.91 | v27.94,31.75 27.94,5.44 X2.2

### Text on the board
tNames: Bank 1 | 1 | 4 | NC | COM | NO | NC | COM | NO | NC | COM | NO | NC | COM | NO | GP7 | GND | GP6 | GP5 | A0 | A1 | GND | A2 | Address | GP4 | SC | MCP23008 | ANSIO4R4G5V1 | SCL | SDA | +5V | GND | REV.A | 2016 ControlEverything.com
